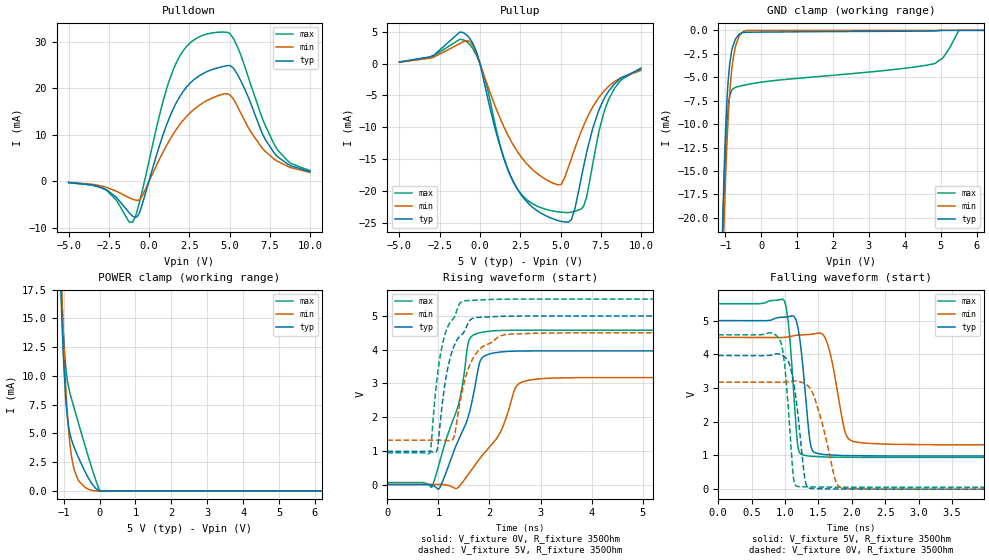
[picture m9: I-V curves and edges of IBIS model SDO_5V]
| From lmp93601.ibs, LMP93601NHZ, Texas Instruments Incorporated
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|   Model SDO_5V
[Model]   SDO_5V
Model_type   3-state
Polarity   Non-Inverting
Vmeas = 2.5
Vref = 5
Cref = 15pF
Rref = 350
|   typ   min   max
|   (nom PVT)   (fast PVT)   (slow PVT)
C_comp   0.1088p   0.1019p   0.1174p
|C_comp (ON state)   0.1088p   0.1019p   0.1174p
|C_comp (OFF state)   0.1091p   0.1021p   0.1180p
[Voltage Range]   5   4.5   5.5
[Temperature Range]   27   125   -25
[Pullup Reference]   5   4.5   5.5
[Pulldown Reference]   0   0   0
[Power Clamp Reference]   5   4.5   5.5
[GND Clamp Reference]   0   0   0
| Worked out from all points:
|   slope of the pulldown table from 0 to 0.75 V, typ, clamps not added: 86.7 ohm
|   slope of the pullup table from 0 to 0.75 V, typ, clamps not added: 90.4 ohm
|   GND clamp passes 1 mA (typ) near -0.72 V on its own axis
|   POWER clamp passes 1 mA (typ) near -0.29 V on its own axis
|   falling waveform, V_fixture 5V, R_fixture 350Ohm: 20-80 % time 115ps typ, 174ps min, 99.1ps max; typ from 5 V to 0.984 V
|   rising waveform, V_fixture 0V, R_fixture 350Ohm: 20-80 % time 492ps typ, 691ps min, 457ps max; typ from 0 V to 3.96 V
|   rising waveform, V_fixture 5V, R_fixture 350Ohm: 20-80 % time 302ps typ, 357ps min, 267ps max; typ from 0.984 V to 5 V
|   falling waveform, V_fixture 0V, R_fixture 350Ohm: 20-80 % time 139ps typ, 239ps min, 105ps max; typ from 3.96 V to 0 V
[Pulldown]
|   Voltage   I(typ)   I(min)   I(max)
-5V       -310.7uA   -263uA     -328uA
-2.705V   -1.781mA   -1.295mA   -1.875mA
-1.04V    -7.512mA   -3.888mA   -8.844mA
-620mV    -6.945mA   -4.052mA   -4.786mA
850mV     9.861mA    6.176mA    17.02mA
1.63V     16.5mA     10.84mA    25.07mA
2.74V     21.72mA    15.32mA    30.31mA
4.42V     24.53mA    18.55mA    32.07mA
5.305V    23.94mA    17.22mA    30.2mA
6.985V    10.52mA    7.234mA    13.87mA
7.99V     5.196mA    4.213mA    6.616mA
9.985V    2.046mA    1.871mA    2.241mA
[GND Clamp]
|   Voltage   I(typ)   I(min)   I(max)
-5V       -931.3mA   -842.1mA   -991.2mA
-1.085V   -21.97mA   -26.76mA   -24.12mA
-1.07V    -19.79mA   -24.75mA   -21.84mA
-1.04V    -15.8mA    -20.95mA   -17.72mA
-995mV    -10.81mA   -15.88mA   -12.83mA
-950mV    -7.122mA   -11.64mA   -9.557mA
-830mV    -2.343mA   -4.484mA   -6.446mA
-710mV    -891.7uA   -1.599mA   -6.072mA
-500mV    -226.9uA   -118.3uA   -5.866mA
4.81V     -74.68uA   0A         -3.564mA
5.515V    0A         0A         0A
9.985V    0A         0A         0A
[Pullup]
|   Voltage   I(typ)   I(min)   I(max)
-5V       275.9uA    245.3uA    246.7uA
-830mV    4.53mA     3.62mA     3.473mA
40mV      -428uA     -294.2uA   -285uA
1.06V     -11.35mA   -7.421mA   -10.89mA
2.11V     -18.75mA   -12.98mA   -18.83mA
4.495V    -24.38mA   -18.76mA   -23.16mA
5.47V     -24.95mA   -16.42mA   -23.44mA
5.89V     -22.81mA   -13.33mA   -23.22mA
6.445V    -16.01mA   -9.663mA   -22.36mA
7.675V    -5.656mA   -4.373mA   -7.832mA
8.68V     -2.411mA   -2.308mA   -2.794mA
9.985V    -817.7uA   -1.073mA   -677.5uA
[POWER Clamp]
|   Voltage   I(typ)   I(min)   I(max)
-5V       603mA      546mA      638.9mA
-1.085V   17.95mA    19.97mA    19.86mA
-1.07V    16.54mA    18.6mA     18.44mA
-1.055V   15.21mA    17.28mA    17.12mA
-995mV    10.72mA    12.48mA    12.96mA
-935mV    7.67mA     8.596mA    10.52mA
-860mV    5.551mA    5.15mA     8.976mA
-785mV    4.483mA    3.063mA    8.035mA
-590mV    2.912mA    936.9uA    5.902mA
-245mV    774.2uA    70.19uA    2.274mA
25mV      0A         0A         0A
9.985V    0A         0A         0A
[Ramp]
R_load = 350
|   typ   min   max
dV/dt_r   2.3782/4.92789e-10   1.90392/6.90552e-10   2.71293/4.57172e-10
dV/dt_f   2.40979/1.14784e-10   1.91138/1.73934e-10   2.73551/9.90395e-11
[Falling Waveform]
V_fixture = 5V
V_fixture_min = 4.5V
V_fixture_max = 5.5V
R_fixture = 350Ohm
C_fixture = 0F
|   Time   V(typ)   V(min)   V(max)
0s        5V         4.5V       5.5V
993.4ps   5.104V     4.503V     5.576V
1.066ns   5.122V     4.52V      4.609V
1.19ns    4.822V     4.568V     1.312V
1.327ns   2.325V     4.582V     990.8mV
1.422ns   1.119V     4.602V     971.1mV
1.646ns   1.019V     4.248V     950.9mV
1.916ns   995.7mV    1.604V     946mV
2.126ns   991.9mV    1.38V      942.2mV
14ns      983.7mV    1.314V     940.8mV
[Rising Waveform]
V_fixture = 0V
V_fixture_min = 0V
V_fixture_max = 0V
R_fixture = 350Ohm
C_fixture = 0F
|   Time   V(typ)   V(min)   V(max)
0s        12.48nV    18.07nV    56.65mV
871.7ps   -20.77mV   230uV      -75.45mV
1.026ns   -101mV     270.6uV    675mV
1.407ns   1.365V     -57.25mV   2.448V
1.59ns    2.045V     310.2mV    4.236V
1.794ns   3.533V     734.6mV    4.496V
2.209ns   3.929V     1.538V     4.567V
2.538ns   3.958V     2.936V     4.577V
2.873ns   3.963V     3.118V     4.577V
14ns      3.964V     3.173V     4.578V
[Rising Waveform]
V_fixture = 5V
V_fixture_min = 4.5V
V_fixture_max = 5.5V
R_fixture = 350Ohm
C_fixture = 0F
|   Time   V(typ)   V(min)   V(max)
0s        983.7mV    1.314V     940.8mV
834.9ps   978mV      1.315V     935.8mV
978.8ps   1.051V     1.315V     3.215V
1.08ns    2.452V     1.314V     4.165V
1.197ns   3.545V     1.3V       4.721V
1.307ns   4.106V     1.408V     4.953V
1.503ns   4.533V     3.013V     5.445V
1.772ns   4.954V     3.957V     5.469V
2.373ns   4.992V     4.458V     5.497V
14ns      5V         4.5V       5.5V
[Falling Waveform]
|Gnd
V_fixture = 0V
V_fixture_min = 0V
V_fixture_max = 0V
R_fixture = 350Ohm
C_fixture = 0F
|   Time   V(typ)   V(min)   V(max)
0s        3.964V     3.173V     4.578V
922.4ps   3.998V     3.169V     4.432V
993.4ps   3.928V     3.175V     3.715V
1.126ns   3.194V     3.2V       363.3mV
1.19ns    2.263V     3.198V     78.92mV
1.323ns   109mV      3.095V     69.49mV
1.514ns   13.63mV    2.25V      61.98mV
1.756ns   5.632mV    258.3mV    60.07mV
1.891ns   4.507mV    21.09mV    59.01mV
14ns      1.42uV     3.561nV    56.65mV
